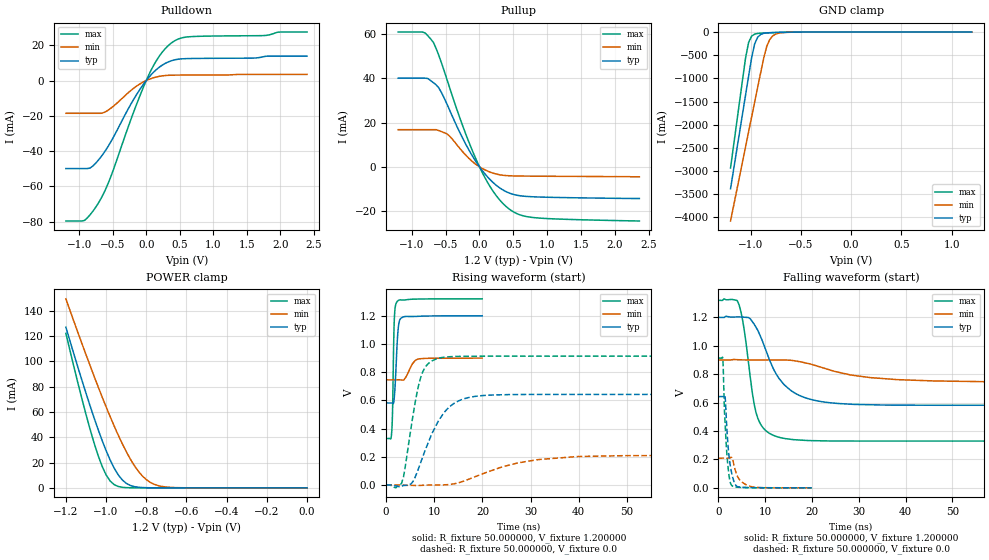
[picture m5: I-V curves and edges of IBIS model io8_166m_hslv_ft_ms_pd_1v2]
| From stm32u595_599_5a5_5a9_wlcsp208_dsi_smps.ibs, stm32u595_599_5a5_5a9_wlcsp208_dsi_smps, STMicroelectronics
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|   Model io8_166m_hslv_ft_ms_pd_1v2
[Model]  io8_166m_hslv_ft_ms_pd_1v2
Model_type I/O
Polarity   Non-Inverting
Enable   Active-Low
Vinl =   0.360000V
Vinh =   0.840000V
Vmeas =  0.600000V
Cref =   50.000000pF
Rref =   100.000000M
Vref =   0.0V
C_comp   3.151700pF   3.087200pF   3.197900pF
[Temperature Range]   25.000000   0.140000k   -40.000000
[Pullup Reference]   1.200000V   0.900000V   1.320000V
[Pulldown Reference]   0.0V   0.0V   0.0V
[POWER Clamp Reference]   1.200000V   0.900000V   1.320000V
[GND Clamp Reference]   0.0V   0.0V   0.0V
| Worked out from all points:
|   slope of the pulldown table from 0 to 0.18 V, typ, clamps not added: 25.4 ohm
|   slope of the pullup table from 0 to 0.18 V, typ, clamps not added: 27.8 ohm
|   GND clamp passes 1 mA (typ) near -0.51 V on its own axis
|   POWER clamp passes 1 mA (typ) near -0.86 V on its own axis
|   rising waveform, R_fixture 50.000000, V_fixture 1.200000: 20-80 % time 558ps typ, 1.42ns min, 312ps max; typ from 0.581 V to 1.2 V
|   rising waveform, R_fixture 50.000000, V_fixture 0.0: 20-80 % time 5.19ns typ, 12.1ns min, 2.72ns max; typ from 0 V to 0.642 V
|   falling waveform, R_fixture 50.000000, V_fixture 1.200000: 20-80 % time 5.91ns typ, 12.5ns min, 2.6ns max; typ from 1.2 V to 0.581 V
|   falling waveform, R_fixture 50.000000, V_fixture 0.0: 20-80 % time 1.03ns typ, 1.72ns min, 824ps max; typ from 0.642 V to 0 V
[Pulldown]
|Voltage   I(typ)   I(min)   I(max)
-1.2V     -49.86mA   -18.57mA   -79.56mA
-920mV    -49.86mA   -18.57mA   -79.19mA
-840mV    -49.6mA    -18.57mA   -76.08mA
-720mV    -45.32mA   -18.57mA   -69.74mA
-560mV    -36.71mA   -16.58mA   -57.44mA
-200mV    -11.43mA   -4.74mA    -19.03mA
0V        -10fA      -600fA     0A
160mV     6.477mA    2.075mA    11.78mA
360mV     10.99mA    2.99mA     20.81mA
480mV     12.07mA    3.054mA    23.53mA
640mV     12.43mA    3.075mA    24.76mA
2.4V      13.79mA    3.434mA    27.44mA
[Pullup]
|Voltage   I(typ)   I(min)   I(max)
-1.2V     40.06mA    16.78mA    60.9mA
-840mV    40.06mA    16.78mA    60.9mA
-680mV    38mA       16.78mA    56.18mA
-600mV    35.64mA    16.38mA    50.28mA
-480mV    28.32mA    14.87mA    39.46mA
-240mV    12.39mA    6.513mA    17.85mA
-40mV     1.772mA    818.2uA    2.67mA
200mV     -7.072mA   -2.851mA   -11mA
440mV     -11.84mA   -4.03mA    -19.1mA
600mV     -13.07mA   -4.154mA   -21.71mA
840mV     -13.59mA   -4.223mA   -23.04mA
2.36V     -14.3mA    -4.5mA     -24.47mA
[GND_clamp]
|Voltage   I(typ)   I(min)   I(max)
-1.2V     -3.379A    -4.076A    -2.932A
-1.05V    -1.35A     -2.47A     -550.7mA
-1.02V    -947.8mA   -2.15A     -221.5mA
-990mV    -552.4mA   -1.829A    -88.45mA
-960mV    -255.3mA   -1.51A     -44.89mA
-930mV    -111.8mA   -1.191A    -30.7mA
-870mV    -28.37mA   -564.6mA   -21.36mA
-840mV    -18.66mA   -309.5mA   -18.51mA
-810mV    -14.08mA   -161.6mA   -15.94mA
-780mV    -11.38mA   -83.33mA   -13.55mA
-600mV    -3.02mA    -4.329mA   -3.104mA
1.2V      30.28uA    18.17uA    37.27uA
[POWER_clamp]
|Voltage   I(typ)   I(min)   I(max)
-1.2V     127mA      149.4mA    122.2mA
-1.12V    84.97mA    114mA      70.27mA
-1.06V    55.51mA    88.42mA    35.67mA
-1.02V    37.63mA    72.04mA    17.17mA
-1V       29.51mA    64.13mA    10.3mA
-960mV    15.69mA    48.99mA    2.571mA
-900mV    3.624mA    28.77mA    182.8uA
-840mV    490.7uA    13.24mA    11.35uA
-800mV    116.8uA    6.532mA    1.77uA
-740mV    13.2uA     1.723mA    109.1nA
-620mV    167.4nA    79.36uA    0A
0V        0A         17.87nA    0A
[Ramp]
| variable   typ   min   max
dV/dt_r  0.38527/5.18683n   0.12539/12.05573n   0.54788/2.70852n
dV/dt_f  0.37097/5.90882n   92.66400m/12.48046n 0.59419/2.58638n
R_load = 50.000000
[Rising Waveform]
R_fixture= 50.000000
V_fixture= 1.200000
V_fixture_min= 0.900000
V_fixture_max= 1.320000
|time   V(typ)   V(min)   V(max)
0s        581.2mV    745.1mV    329.2mV
1.121ns   581.4mV    745.1mV    361mV
1.321ns   579.1mV    745.1mV    514.5mV
1.562ns   585.7mV    745.1mV    1.003V
1.682ns   618.2mV    745.1mV    1.163V
2.242ns   977.1mV    745.2mV    1.299V
2.683ns   1.154V     745.2mV    1.311V
3.564ns   1.191V     743.7mV    1.311V
6.527ns   1.196V     891.4mV    1.318V
19.94ns   1.2V       899.5mV    1.319V
[Rising Waveform]
R_fixture= 50.000000
V_fixture= 0.0
V_fixture_min= 0.0
V_fixture_max= 0.0
|time   V(typ)   V(min)   V(max)
0s        1.941nV    235.2nV    1.147nV
3.203ns   -9.394mV   133.5uV    12.26mV
5.205ns   8.907mV    -3.022mV   413.2mV
7.207ns   162.4mV    -3.183mV   765.6mV
8.809ns   305.5mV    -863.9uV   862.1mV
12.01ns   512.5mV    592.7uV    905.7mV
18.42ns   627.7mV    57.47mV    912.8mV
27.23ns   641.2mV    155.2mV    913.1mV
40.04ns   642mV      201.9mV    913.1mV
199.4ns   642.1mV    209.1mV    913.1mV
[Falling Waveform]
R_fixture= 50.000000
V_fixture= 1.200000
V_fixture_min= 0.900000
V_fixture_max= 1.320000
|time   V(typ)   V(min)   V(max)
0s        1.2V       899.5mV    1.319V
4.004ns   1.203V     901.9mV    1.318V
5.205ns   1.202V     900.4mV    1.171V
7.207ns   1.171V     900.2mV    673.8mV
8.408ns   1.108V     900.2mV    489.4mV
12.01ns   819.9mV    900mV      365.7mV
14.41ns   714.8mV    899.3mV    345.9mV
23.22ns   601.1mV    835.6mV    330.1mV
46.05ns   581.3mV    752.3mV    329.2mV
199.4ns   581.2mV    745.1mV    329.2mV
[Falling Waveform]
R_fixture= 50.000000
V_fixture= 0.0
V_fixture_min= 0.0
V_fixture_max= 0.0
|time   V(typ)   V(min)   V(max)
0s        642.1mV    209.1mV    913.1mV
920.9ps   642.3mV    209.1mV    908.2mV
1.241ns   647.7mV    209.2mV    572.7mV
1.401ns   644.4mV    209.2mV    461.5mV
1.722ns   457mV      209.2mV    271mV
2.202ns   237.5mV    209mV      99.92mV
2.763ns   112.5mV    214.6mV    19.48mV
3.804ns   14.17mV    101.4mV    5.158mV
6.286ns   2.465mV    16.5mV     1.131mV
19.94ns   1.941nV    235.2nV    1.147nV
